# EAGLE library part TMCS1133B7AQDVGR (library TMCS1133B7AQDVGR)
Board Mount Current Sensors +/-1300V reinforced isolation 80ARMS 1M Source: Datasheet
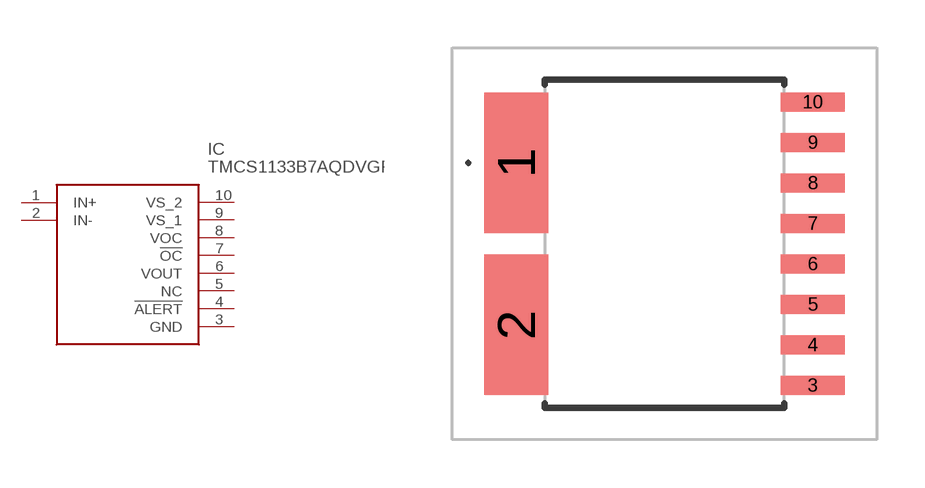
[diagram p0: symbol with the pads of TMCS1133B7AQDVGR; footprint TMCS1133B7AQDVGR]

Designator prefix IC

## TMCS1133B7AQDVGR (Description: Board Mount Current Sensors +/-1300V reinforced isolation 80ARMS 1M; Height: 2.65mm; Manufacturer_Name: Texas Instruments; Manufacturer_Part_Number: TMCS1133B7AQDVGR)  [TMCS1133B7AQDVGR]
1  IN+
2  IN-
3  GND
4  !ALERT
5  NC  nc
6  VOUT
7  !OC
8  VOC
9  VS_1
10  VS_2

## Footprint TMCS1133B7AQDVGR (pad centres in mm)
DVG0010A_2026
smd 2 x 4.41: 1 -4.65,2.54; 2 -4.65,-2.54
smd 2 x 0.6: 3 4.65,-4.445; 4 4.65,-3.175; 5 4.65,-1.905; 6 4.65,-0.635; 7 4.65,0.635; 8 4.65,1.905; 9 4.65,3.175; 10 4.65,4.445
